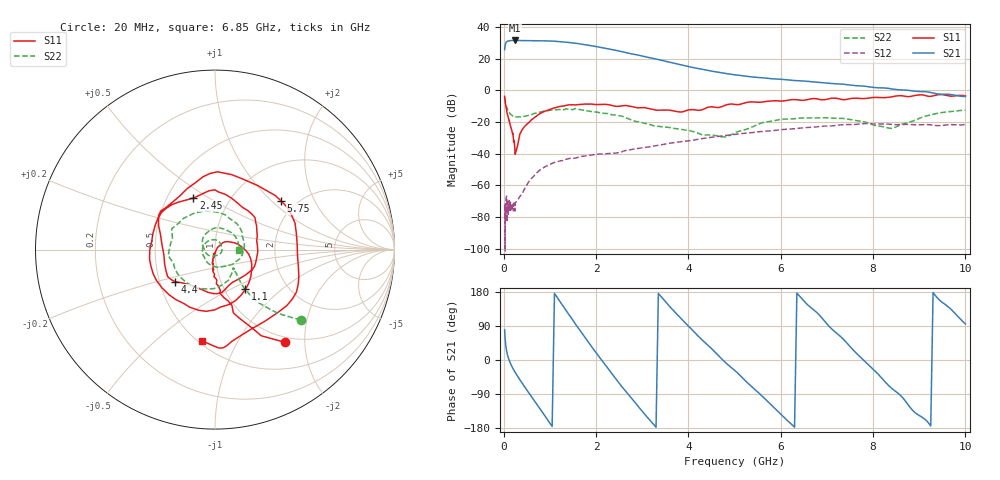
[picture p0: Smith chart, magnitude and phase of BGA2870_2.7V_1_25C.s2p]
#  HZ  S  RI  R  50.0000
! Rohde & Schwarz ZVA/B
! Temperature 25C
! Device number 1
! Measured Vcc 2.700000
! Measured Icc 0.017800
! DeltaGain  -0.063561  3dBBWHighMHz 1897.83  3dBBWLowMHz 29.13
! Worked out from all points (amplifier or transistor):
!   242 points, 20 MHz to 10 GHz, reference 50 ohm
!   highest |S21| = 31.5 dB at 245 MHz (marker M1)
!   |S21| within 3 dB of that: 31.32 MHz to 1.826 GHz (1.795 GHz wide, 193 % of centre)
!   unconditionally stable (mu >= 1): start of sweep to end of sweep
!   at 220 MHz: K = 53.83, MAG = 31.6 dB, |S12| = -72.4 dB
!   at 4 GHz: K = 3.39, MAG = 15.3 dB, |S12| = -32.0 dB
!   at 10 GHz: K = 5.00, MAG = -1.1 dB, |S12| = -21.6 dB
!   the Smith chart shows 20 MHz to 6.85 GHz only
!   S11 on the Smith chart (normalised r, x): 20 MHz: 0.91, -1.61; 1.1 GHz: 1.25, -0.60; 2.45 GHz: 0.67, +0.43; 4.4 GHz: 0.60, -0.23; 5.75 GHz: 1.67, +1.15; 6.85 GHz: 0.52, -0.72
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2e7  0.3892 -0.5164  3.506 19.01  0.000223 -8.02e-05  0.4781 -0.3922
5e7  0.072 -0.2846  26.88 17.96  0.000391 -1.89e-05  0.2185 -0.2774
9e7  0.00122 -0.1574  35.66 6.094  -0.000166 -6.16e-05  0.1447 -0.1855
2.45e8  0.00319 -0.0101  32.1 -19.94  9.51e-05 0.000121  0.1054 -0.1056
4.5e8  0.0567 0.0438  12.77 -35.22  -0.000123 0.000757  0.1006 -0.1129
6.5e8  0.1287 0.0297  -9.619 -36.05  0.000119 0.00194  0.0809 -0.1666
9e8  0.205 -0.0825  -31.41 -18.93  0.00258 0.00291  -0.0345 -0.2196
1.1e9  0.1699 -0.2215  -35.66 2.685  0.00496 0.00186  -0.1588 -0.1845
1.4e9  -0.0487 -0.3438  -17.36 27.77  0.00668 -0.00178  -0.2536 0.00614
1.7e9  -0.2951 -0.2133  10.03 26.78  0.00561 -0.00608  -0.147 0.188
2.05e9  -0.3457 0.09  23.11 4.544  0.00131 -0.00955  0.0579 0.1935
2.45e9  -0.1204 0.2874  10.85 -14.57  -0.00457 -0.00946  0.1643 0.0229
2.95e9  0.1823 0.2178  -7.789 -9.966  -0.014 -0.00503  0.018 -0.0991
3.35e9  0.2365 0.0199  -9.375 0.7287  -0.0177 0.00524  -0.0653 -0.0334
3.8e9  0.1245 -0.1681  -2.758 6.015  -0.0107 0.0209  -0.0331 0.05
4.4e9  -0.2234 -0.1783  3.26 2.869  0.0173 0.0262  0.0389 0.00516
5.05e9  -0.2411 0.2609  2.572 -1.63  0.0403 -0.0101  -0.037 -0.0312
5.75e9  0.3684 0.271  -0.937 -2.182  -0.00188 -0.0524  -0.0462 0.0926
6.7e9  0.046 -0.5472  -1.273 1.338  -0.0662 0.0188  0.1308 0.0302
6.85e9  -0.0744 -0.5068  -0.8071 1.589  -0.0619 0.037  0.1354 -0.00241
8.35e9  0.2105 0.5671  0.4119 -1.07  0.0779 -0.0351  -0.00784 -0.0637
1e10  -0.1648 -0.6529  -0.0573 0.6379  -0.0827 0.0122  -0.2365 -0.00147
